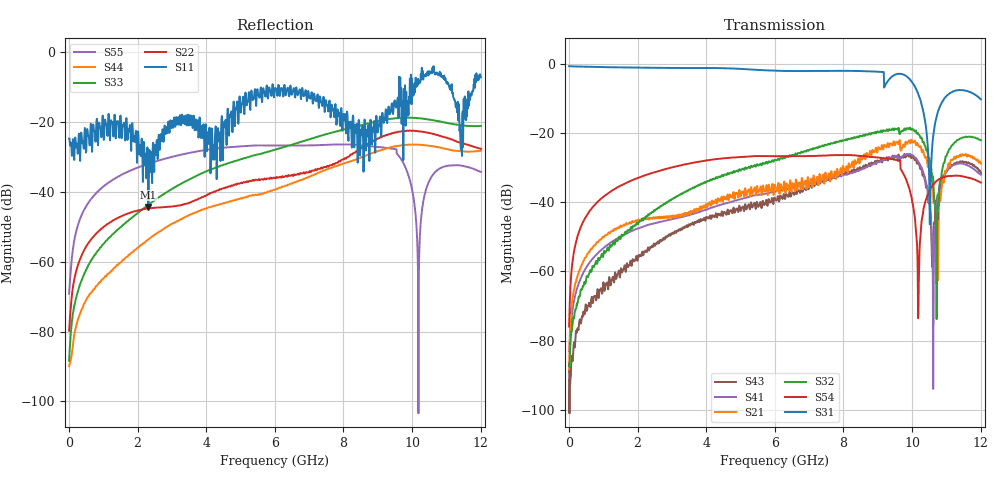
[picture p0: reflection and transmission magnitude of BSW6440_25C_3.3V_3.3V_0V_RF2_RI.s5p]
!	Test time	=	2022-08-08 18:05
!	Product	=	BSW6440
!	Temp	=	25C
!	VDD	=	3.3
!	Control_High	=	3.3
!	Control_Low	=	0
!	Logic	=	RF2
!	Porrt1	=	RFC
!	Porrt2	=	RF1
!	Porrt3	=	RF2
!	Porrt4	=	RF3
!	Porrt5	=	RF4
!	V1(LS)	=	0
!	V2(CTRL)	=	X
!	V3	=	X
!	V4	=	X
#	Hz	S	RI	R	50
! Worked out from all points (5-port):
!   1201 points, 5 MHz to 12.01 GHz, reference 50 ohm
!   strongest paths, dB at 5 MHz, 3.005 GHz, 6.005 GHz, 9.005 GHz, 12.01 GHz:
!     S31: -0.6, -1.2, -2.0, -2.3, -10.2
!     S54: -76.0, -29.9, -26.7, -27.0, -34.3
!     S32: -87.2, -39.1, -27.8, -19.6, -22.1
!     S21: -88.4, -44.5, -35.0, -24.4, -28.8
!     S41: -83.1, -44.9, -37.0, -28.4, -32.0
!     S43: -86.8, -49.2, -39.0, -28.2, -31.6
!   lowest |S11| = -44.3 dB at 2.315 GHz (marker M1), VSWR 1.01, Z = 50.2 + j0.572 ohm
!   |S11| at or under -10 dB: start of sweep to 5.754 GHz; 6.465 GHz to 9.619 GHz (3.154 GHz wide, 39.2 % of centre); 11.16 GHz to 11.79 GHz (630.5 MHz wide, 5.49 % of centre)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
